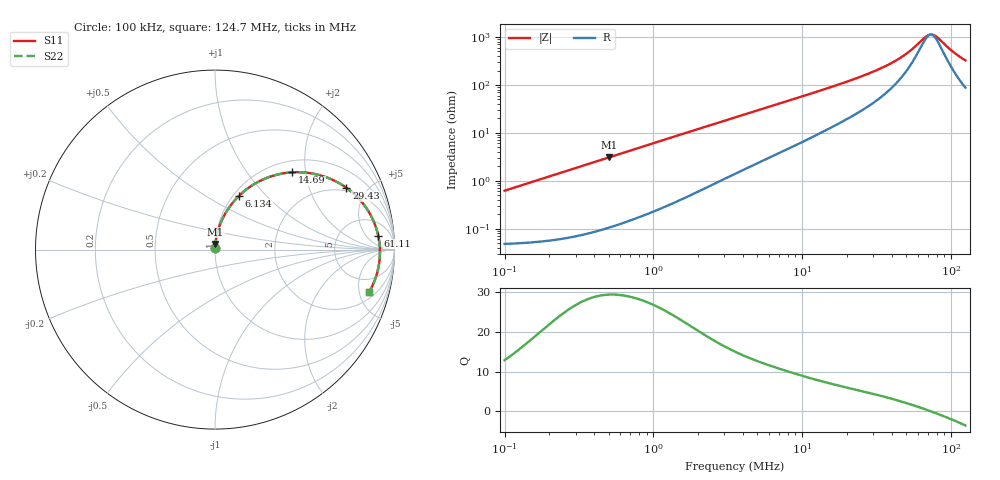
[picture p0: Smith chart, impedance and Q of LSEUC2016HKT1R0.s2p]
! LSEUC2016HKT1R0  S-PARAMETER MODEL  ( General Type )
! Model Generated by TAIYO YUDEN Corporation (http://www.ty-top.com)
! Version 1.0
! TAIYO YUDEN Control No. 211126
! Copyright(c) 2021 TAIYO YUDEN CO.,LTD. All Rights Reserved.
! Product Description (link to TY-COMPAS)
! https://ds.yuden.co.jp/TYCOMPAS/or/detail?pn=LSEUC2016HKT1R0M&u=M
! Products Name : Inductors
! Characteristics :
!  Inductance : 1.0 uH , SRF(min) : -Hz , DC Resistance(max) : 0.05 Ohm
!  Rated Current : Saturation :3200 mA , Temp Rise : 3000 mA (40 degC)
!  Case Size : 2.0 x 1.6 / 0.079 x 0.063 [mm/inch] , Thickness : 0.8 / 0.031 [mm/inch]
!  (Conditions: Temperature = 25 degC , DC Bias Current/Voltage = 0A / 0V)
! External Node Assignments :
!  1  o---GGG---o  2
! GND o---------o GND
! Frequency Range : 0.1MHz  -  124.6553MHz  [ 402 STEP ]
# MHz S RI R 50
! Freq[MHz].  S11 Real  S11 Imag  S21 Real  S21 Imag  S12 Real  S12 Imag  S22 Real  S22 Imag
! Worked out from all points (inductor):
!   401 points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, 100 kHz to 124.7 MHz, reference 50 ohm
!   read as one part in series: L = 982 nH near 103.6 kHz
!   highest Q = 29.4 at 506.1 kHz (marker M1), where L = 976 nH
!   self-resonance near 72.98 MHz
!   S11 on the Smith chart (normalised r, x): 100 kHz: 1.00, +0.01; 6.134 MHz: 1.06, +0.71; 14.69 MHz: 1.23, +1.68; 29.43 MHz: 1.81, +3.61; 61.11 MHz: 12, +11; 124.7 MHz: 2.76, -6.28
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0.1  0.000516 0.00616  0.9995 -0.00616  0.9995 -0.00616  0.000516 0.00616
0.330013  0.00115 0.0203  0.9989 -0.0203  0.9989 -0.0203  0.00115 0.0203
0.506144  0.00201 0.0309  0.998 -0.0309  0.998 -0.0309  0.00201 0.0309
1.089088  0.00685 0.0655  0.9932 -0.0655  0.9932 -0.0655  0.00685 0.0655
2.032066  0.0205 0.1189  0.9795 -0.1189  0.9795 -0.1189  0.0205 0.1189
3.530656  0.054 0.1952  0.946 -0.1952  0.946 -0.1952  0.054 0.1952
6.134412  0.134 0.2998  0.866 -0.2998  0.866 -0.2998  0.134 0.2998
8.454345  0.2164 0.3638  0.7836 -0.3638  0.7836 -0.3638  0.2164 0.3638
11.65164  0.3305 0.4135  0.6695 -0.4135  0.6695 -0.4135  0.3305 0.4135
14.68918  0.4289 0.4304  0.5711 -0.4304  0.5711 -0.4304  0.4289 0.4304
20.60838  0.5824 0.415  0.4176 -0.415  0.4176 -0.415  0.5824 0.415
29.43265  0.7318 0.3448  0.2682 -0.3448  0.2682 -0.3448  0.7318 0.3448
38.45196  0.821 0.2615  0.179 -0.2615  0.179 -0.2615  0.821 0.2615
49.34786  0.8799 0.1668  0.1201 -0.1668  0.1201 -0.1668  0.8799 0.1668
61.11385  0.9095 0.0774  0.0905 -0.0774  0.0905 -0.0774  0.9095 0.0774
69.23323  0.9176 0.0232  0.0824 -0.0232  0.0824 -0.0232  0.9176 0.0232
73.03524  0.9189 -0.000341  0.0811 0.000341  0.0811 0.000341  0.9189 -0.000341
75.68521  0.9191 -0.0161  0.0809 0.0161  0.0809 0.0161  0.9191 -0.0161
81.27708  0.9178 -0.0477  0.0822 0.0477  0.0822 0.0477  0.9178 -0.0477
104.3081  0.8946 -0.1581  0.1054 0.1581  0.1054 0.1581  0.8946 -0.1581
118.1661  0.8719 -0.212  0.1281 0.212  0.1281 0.212  0.8719 -0.212
124.6553  0.8598 -0.2344  0.1402 0.2344  0.1402 0.2344  0.8598 -0.2344
